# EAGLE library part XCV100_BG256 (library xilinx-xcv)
xcv100_bg256_1532 edit this description Auto generated by make-symbol-device-package-bsdl.ulp Rev. 25 Source: xcv100_bg256_1532.bsd
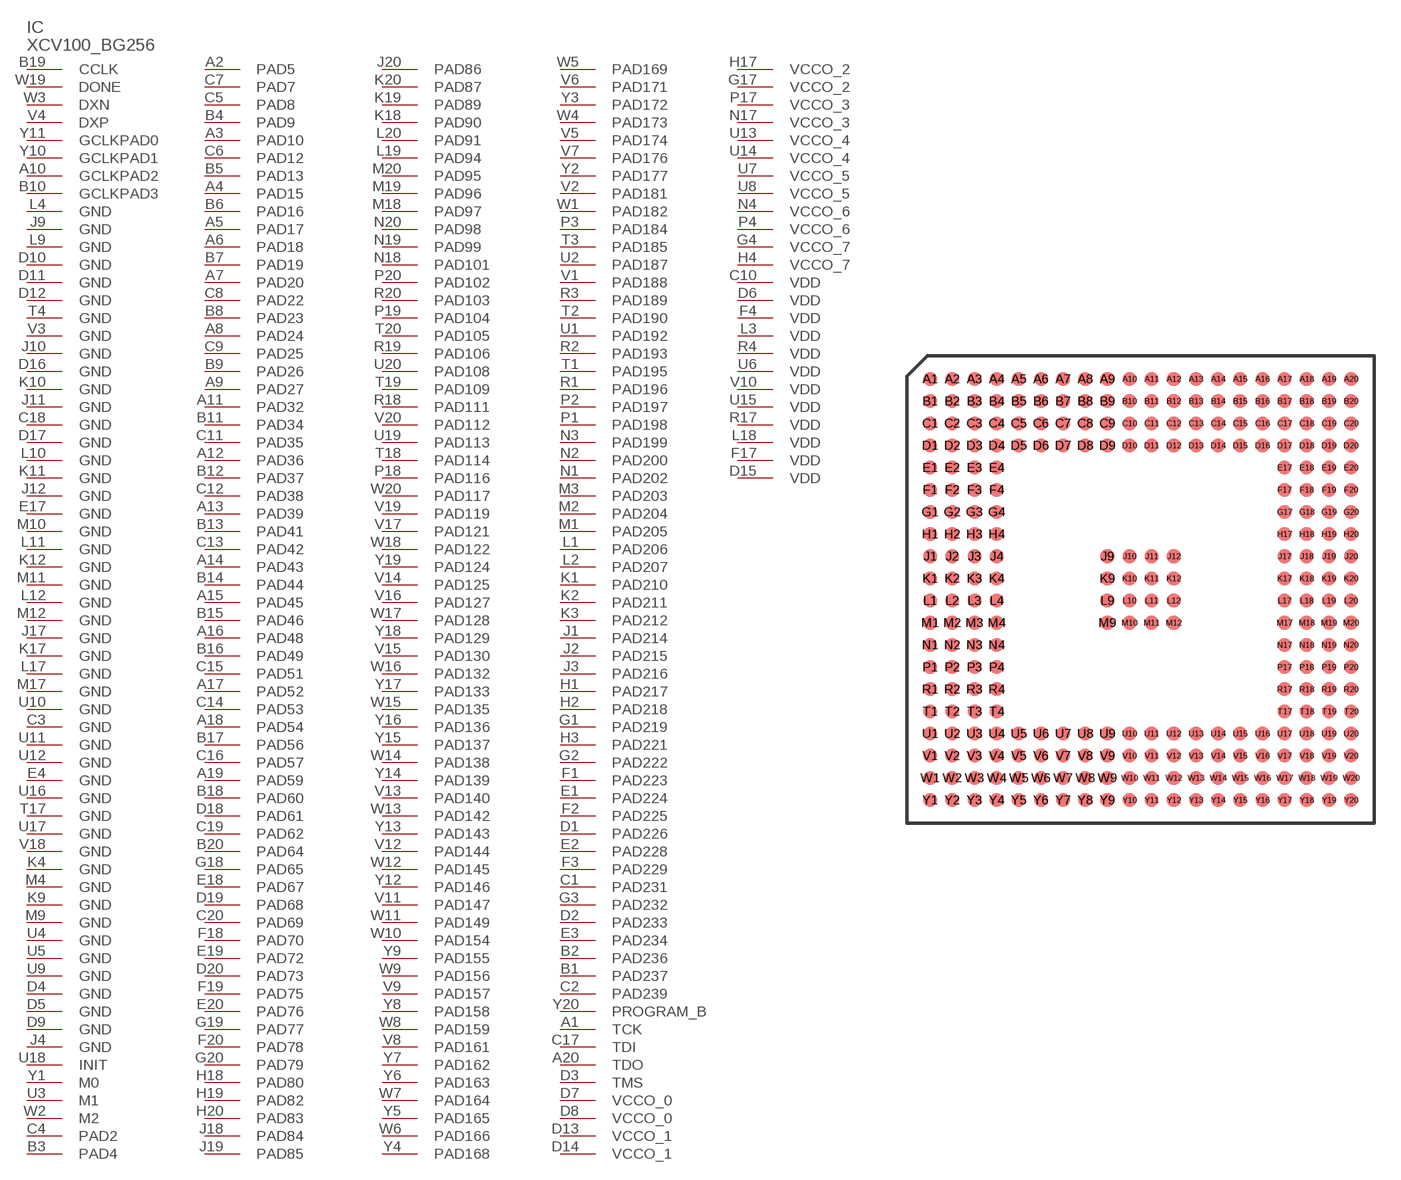
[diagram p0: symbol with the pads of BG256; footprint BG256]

Designator prefix IC

## XCV100_BG256 (OC_FARNELL: unknown; OC_NEWARK: unknown)  [BG256]
A1  TCK  in
A2  PAD5
A3  PAD10
A4  PAD15
A5  PAD17
A6  PAD18
A7  PAD20
A8  PAD24
A9  PAD27
A10  GCLKPAD2  in
A11  PAD32
A12  PAD36
A13  PAD39
A14  PAD43
A15  PAD45
A16  PAD48
A17  PAD52
A18  PAD54
A19  PAD59
A20  TDO  out
B1  PAD237
B2  PAD236
B3  PAD4
B4  PAD9
B5  PAD13
B6  PAD16
B7  PAD19
B8  PAD23
B9  PAD26
B10  GCLKPAD3  in
B11  PAD34
B12  PAD37
B13  PAD41
B14  PAD44
B15  PAD46
B16  PAD49
B17  PAD56
B18  PAD60
B19  CCLK
B20  PAD64
C1  PAD231
C2  PAD239
C3  GND  pwr
C4  PAD2
C5  PAD8
C6  PAD12
C7  PAD7
C8  PAD22
C9  PAD25
C10  VDD  pwr
C11  PAD35
C12  PAD38
C13  PAD42
C14  PAD53
C15  PAD51
C16  PAD57
C17  TDI  in
C18  GND  pwr
C19  PAD62
C20  PAD69
D1  PAD226
D2  PAD233
D3  TMS  in
D4  GND  pwr
D5  GND  pwr
D6  VDD  pwr
D7  VCCO_0  pwr
D8  VCCO_0  pwr
D9  GND  pwr
D10  GND  pwr
D11  GND  pwr
D12  GND  pwr
D13  VCCO_1  pwr
D14  VCCO_1  pwr
D15  VDD  pwr
D16  GND  pwr
D17  GND  pwr
D18  PAD61
D19  PAD68
D20  PAD73
E1  PAD224
E2  PAD228
E3  PAD234
E4  GND  pwr
E17  GND  pwr
E18  PAD67
E19  PAD72
E20  PAD76
F1  PAD223
F2  PAD225
F3  PAD229
F4  VDD  pwr
F17  VDD  pwr
F18  PAD70
F19  PAD75
F20  PAD78
G1  PAD219
G2  PAD222
G3  PAD232
G4  VCCO_7  pwr
G17  VCCO_2  pwr
G18  PAD65
G19  PAD77
G20  PAD79
H1  PAD217
H2  PAD218
H3  PAD221
H4  VCCO_7  pwr
H17  VCCO_2  pwr
H18  PAD80
H19  PAD82
H20  PAD83
J1  PAD214
J2  PAD215
J3  PAD216
J4  GND  pwr
J9  GND  pwr
J10  GND  pwr
J11  GND  pwr
J12  GND  pwr
J17  GND  pwr
J18  PAD84
J19  PAD85
J20  PAD86
K1  PAD210
K2  PAD211
K3  PAD212
K4  GND  pwr
K9  GND  pwr
K10  GND  pwr
K11  GND  pwr
K12  GND  pwr
K17  GND  pwr
K18  PAD90
K19  PAD89
K20  PAD87
L1  PAD206
L2  PAD207
L3  VDD  pwr
L4  GND  pwr
L9  GND  pwr
L10  GND  pwr
L11  GND  pwr
L12  GND  pwr
L17  GND  pwr
L18  VDD  pwr
L19  PAD94
L20  PAD91
M1  PAD205
M2  PAD204
M3  PAD203
M4  GND  pwr
M9  GND  pwr
M10  GND  pwr
M11  GND  pwr
M12  GND  pwr
M17  GND  pwr
M18  PAD97
M19  PAD96
M20  PAD95
N1  PAD202
N2  PAD200
N3  PAD199
N4  VCCO_6  pwr
N17  VCCO_3  pwr
N18  PAD101
N19  PAD99
N20  PAD98
P1  PAD198
P2  PAD197
P3  PAD184
P4  VCCO_6  pwr
P17  VCCO_3  pwr
P18  PAD116
P19  PAD104
P20  PAD102
R1  PAD196
R2  PAD193
R3  PAD189
R4  VDD  pwr
R17  VDD  pwr
R18  PAD111
R19  PAD106
R20  PAD103
T1  PAD195
T2  PAD190
T3  PAD185
T4  GND  pwr
T17  GND  pwr
T18  PAD114
T19  PAD109
T20  PAD105
U1  PAD192
U2  PAD187
U3  M1  in
U4  GND  pwr
U5  GND  pwr
U6  VDD  pwr
U7  VCCO_5  pwr
U8  VCCO_5  pwr
U9  GND  pwr
U10  GND  pwr
U11  GND  pwr
U12  GND  pwr
U13  VCCO_4  pwr
U14  VCCO_4  pwr
U15  VDD  pwr
U16  GND  pwr
U17  GND  pwr
U18  INIT
U19  PAD113
U20  PAD108
V1  PAD188
V2  PAD181
V3  GND  pwr
V4  DXP  pas
V5  PAD174
V6  PAD171
V7  PAD176
V8  PAD161
V9  PAD157
V10  VDD  pwr
V11  PAD147
V12  PAD144
V13  PAD140
V14  PAD125
V15  PAD130
V16  PAD127
V17  PAD121
V18  GND  pwr
V19  PAD119
V20  PAD112
W1  PAD182
W2  M2  in
W3  DXN  pas
W4  PAD173
W5  PAD169
W6  PAD166
W7  PAD164
W8  PAD159
W9  PAD156
W10  PAD154
W11  PAD149
W12  PAD145
W13  PAD142
W14  PAD138
W15  PAD135
W16  PAD132
W17  PAD128
W18  PAD122
W19  DONE
W20  PAD117
Y1  M0  in
Y2  PAD177
Y3  PAD172
Y4  PAD168
Y5  PAD165
Y6  PAD163
Y7  PAD162
Y8  PAD158
Y9  PAD155
Y10  GCLKPAD1  in
Y11  GCLKPAD0  in
Y12  PAD146
Y13  PAD143
Y14  PAD139
Y15  PAD137
Y16  PAD136
Y17  PAD133
Y18  PAD129
Y19  PAD124
Y20  PROGRAM_B  in

## Footprint BG256 (pad centres in mm)
xcv100_bg256_1532 edit this description Auto generated by make-symbol-device-package-bsdl.ulp Rev. 25 Source: xcv100_bg256_1532.bsd
smd 0.8 x 0.8: A1 -12.065,12.065; A2 -10.795,12.065; A3 -9.525,12.065; A4 -8.255,12.065; A5 -6.985,12.065; A6 -5.715,12.065; A7 -4.445,12.065; A8 -3.175,12.065; A9 -1.905,12.065; A10 -0.635,12.065; A11 0.635,12.065; A12 1.905,12.065; A13 3.175,12.065; A14 4.445,12.065; A15 5.715,12.065; A16 6.985,12.065; A17 8.255,12.065; A18 9.525,12.065; A19 10.795,12.065; A20 12.065,12.065; B1 -12.065,10.795; B2 -10.795,10.795; B3 -9.525,10.795; B4 -8.255,10.795; B5 -6.985,10.795; B6 -5.715,10.795; B7 -4.445,10.795; B8 -3.175,10.795; B9 -1.905,10.795; B10 -0.635,10.795; B11 0.635,10.795; B12 1.905,10.795; B13 3.175,10.795; B14 4.445,10.795; B15 5.715,10.795; B16 6.985,10.795; B17 8.255,10.795; B18 9.525,10.795; B19 10.795,10.795; B20 12.065,10.795; C1 -12.065,9.525; C2 -10.795,9.525; C3 -9.525,9.525; C4 -8.255,9.525; C5 -6.985,9.525; C6 -5.715,9.525; C7 -4.445,9.525; C8 -3.175,9.525; C9 -1.905,9.525; C10 -0.635,9.525; C11 0.635,9.525; C12 1.905,9.525; C13 3.175,9.525; C14 4.445,9.525; C15 5.715,9.525; C16 6.985,9.525; C17 8.255,9.525; C18 9.525,9.525; C19 10.795,9.525; C20 12.065,9.525; D1 -12.065,8.255; D2 -10.795,8.255; D3 -9.525,8.255; D4 -8.255,8.255; D5 -6.985,8.255; D6 -5.715,8.255; D7 -4.445,8.255; D8 -3.175,8.255; D9 -1.905,8.255; D10 -0.635,8.255; D11 0.635,8.255; D12 1.905,8.255; D13 3.175,8.255; D14 4.445,8.255; D15 5.715,8.255; D16 6.985,8.255; D17 8.255,8.255; D18 9.525,8.255; D19 10.795,8.255; D20 12.065,8.255; E1 -12.065,6.985; E2 -10.795,6.985; E3 -9.525,6.985; E4 -8.255,6.985; E17 8.255,6.985; E18 9.525,6.985; E19 10.795,6.985; E20 12.065,6.985; F1 -12.065,5.715; F2 -10.795,5.715; F3 -9.525,5.715; F4 -8.255,5.715; F17 8.255,5.715; F18 9.525,5.715; F19 10.795,5.715; F20 12.065,5.715; G1 -12.065,4.445; G2 -10.795,4.445; G3 -9.525,4.445; G4 -8.255,4.445; G17 8.255,4.445; G18 9.525,4.445; G19 10.795,4.445; G20 12.065,4.445; H1 -12.065,3.175; H2 -10.795,3.175; H3 -9.525,3.175; H4 -8.255,3.175; H17 8.255,3.175; H18 9.525,3.175; H19 10.795,3.175; H20 12.065,3.175; J1 -12.065,1.905; J2 -10.795,1.905; J3 -9.525,1.905; J4 -8.255,1.905; J9 -1.905,1.905; J10 -0.635,1.905; J11 0.635,1.905; J12 1.905,1.905; J17 8.255,1.905; J18 9.525,1.905; J19 10.795,1.905; J20 12.065,1.905; K1 -12.065,0.635; K2 -10.795,0.635; K3 -9.525,0.635; K4 -8.255,0.635; K9 -1.905,0.635; K10 -0.635,0.635; K11 0.635,0.635; K12 1.905,0.635; K17 8.255,0.635; K18 9.525,0.635; K19 10.795,0.635; K20 12.065,0.635; L1 -12.065,-0.635; L2 -10.795,-0.635; L3 -9.525,-0.635; L4 -8.255,-0.635; L9 -1.905,-0.635; L10 -0.635,-0.635; L11 0.635,-0.635; L12 1.905,-0.635; L17 8.255,-0.635; L18 9.525,-0.635; L19 10.795,-0.635; L20 12.065,-0.635; M1 -12.065,-1.905; M2 -10.795,-1.905; M3 -9.525,-1.905; M4 -8.255,-1.905; M9 -1.905,-1.905; M10 -0.635,-1.905; M11 0.635,-1.905; M12 1.905,-1.905; M17 8.255,-1.905; M18 9.525,-1.905; M19 10.795,-1.905; M20 12.065,-1.905; N1 -12.065,-3.175; N2 -10.795,-3.175; N3 -9.525,-3.175; N4 -8.255,-3.175; N17 8.255,-3.175; N18 9.525,-3.175; N19 10.795,-3.175; N20 12.065,-3.175; P1 -12.065,-4.445; P2 -10.795,-4.445; P3 -9.525,-4.445; P4 -8.255,-4.445; P17 8.255,-4.445; P18 9.525,-4.445; P19 10.795,-4.445; P20 12.065,-4.445; R1 -12.065,-5.715; R2 -10.795,-5.715; R3 -9.525,-5.715; R4 -8.255,-5.715; R17 8.255,-5.715; R18 9.525,-5.715; R19 10.795,-5.715; R20 12.065,-5.715; T1 -12.065,-6.985; T2 -10.795,-6.985; T3 -9.525,-6.985; T4 -8.255,-6.985; T17 8.255,-6.985; T18 9.525,-6.985; T19 10.795,-6.985; T20 12.065,-6.985; U1 -12.065,-8.255; U2 -10.795,-8.255; U3 -9.525,-8.255; U4 -8.255,-8.255; U5 -6.985,-8.255; U6 -5.715,-8.255; U7 -4.445,-8.255; U8 -3.175,-8.255; U9 -1.905,-8.255; U10 -0.635,-8.255; U11 0.635,-8.255; U12 1.905,-8.255; U13 3.175,-8.255; U14 4.445,-8.255; U15 5.715,-8.255; U16 6.985,-8.255; U17 8.255,-8.255; U18 9.525,-8.255; U19 10.795,-8.255; U20 12.065,-8.255; V1 -12.065,-9.525; V2 -10.795,-9.525; V3 -9.525,-9.525; V4 -8.255,-9.525; V5 -6.985,-9.525; V6 -5.715,-9.525; V7 -4.445,-9.525; V8 -3.175,-9.525; V9 -1.905,-9.525; V10 -0.635,-9.525; V11 0.635,-9.525; V12 1.905,-9.525; V13 3.175,-9.525; V14 4.445,-9.525; V15 5.715,-9.525; V16 6.985,-9.525; V17 8.255,-9.525; V18 9.525,-9.525; V19 10.795,-9.525; V20 12.065,-9.525; W1 -12.065,-10.795; W2 -10.795,-10.795; W3 -9.525,-10.795; W4 -8.255,-10.795; W5 -6.985,-10.795; W6 -5.715,-10.795; W7 -4.445,-10.795; W8 -3.175,-10.795; W9 -1.905,-10.795; W10 -0.635,-10.795; W11 0.635,-10.795; W12 1.905,-10.795; W13 3.175,-10.795; W14 4.445,-10.795; W15 5.715,-10.795; W16 6.985,-10.795; W17 8.255,-10.795; W18 9.525,-10.795; W19 10.795,-10.795; W20 12.065,-10.795; Y1 -12.065,-12.065; Y2 -10.795,-12.065; Y3 -9.525,-12.065; Y4 -8.255,-12.065; Y5 -6.985,-12.065; Y6 -5.715,-12.065; Y7 -4.445,-12.065; Y8 -3.175,-12.065; Y9 -1.905,-12.065; Y10 -0.635,-12.065; Y11 0.635,-12.065; Y12 1.905,-12.065; Y13 3.175,-12.065; Y14 4.445,-12.065; Y15 5.715,-12.065; Y16 6.985,-12.065; Y17 8.255,-12.065; Y18 9.525,-12.065; Y19 10.795,-12.065; Y20 12.065,-12.065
